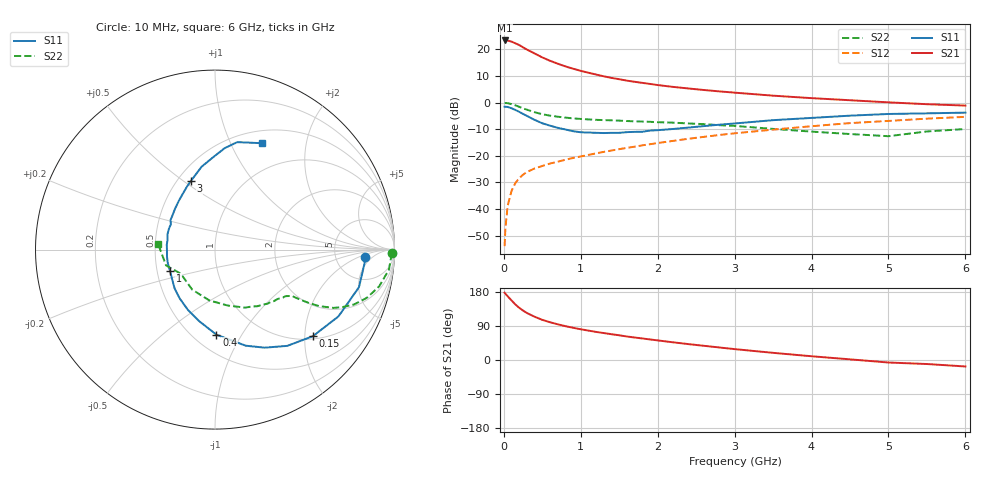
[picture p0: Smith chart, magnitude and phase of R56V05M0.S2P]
! SIEMENS Small Signal Semiconductors
! BFR183
! Si NPN RF Bipolar Junction Transistor in SOT23
! VCE = 6 V  IC = 5 mA
! Common Emitter S-Parameters:  May  1996
# GHz  S  MA  R  50
!  f  S11  S21  S12  S22
! GHz  MAG  ANG  MAG  ANG  MAG  ANG  MAG  ANG
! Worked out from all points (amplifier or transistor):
!   36 points, 10 MHz to 6 GHz, reference 50 ohm
!   highest |S21| = 23.4 dB at 10 MHz (marker M1)
!   |S21| within 3 dB of that: start of sweep to 274.3 MHz
!   unconditionally stable (mu >= 1): 1.052 GHz to 2.66 GHz
!   at 250 MHz: K = 0.42, MSG = 23.9 dB, |S12| = -27.1 dB
!   at 1.4 GHz: K = 1.05, MAG = 12.2 dB, |S12| = -18.0 dB
!   at 6 GHz: K = 0.88, MSG = 2.1 dB, |S12| = -5.4 dB
!   lowest NFmin = 1.15 dB at 450 MHz
!   S11 on the Smith chart (normalised r, x): 10 MHz: 10, -3; 150 MHz: 1.07, -2.20; 400 MHz: 0.64, -0.78; 1 GHz: 0.58, -0.15; 3 GHz: 0.58, +0.53; 6 GHz: 0.65, +1.32
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0.01  0.8377 -2.9  14.73 177.6  0.002 86.8  0.9876 -1.2
0.02  0.8359 -5.7  14.59 175.0  0.0043 83.7  0.982 -2.6
0.05  0.8291 -14.6  14.68 168.1  0.0115 83.2  0.9754 -6.6
0.1  0.7822 -28.4  14.02 157.2  0.0219 76.6  0.9369 -12.7
0.15  0.7281 -41.5  13.01 146.5  0.0308 69.7  0.8877 -17.6
0.2  0.6707 -53.1  12.08 137.8  0.0381 65.5  0.8334 -21.5
0.25  0.6127 -63.1  10.92 130.4  0.0442 61.6  0.7786 -24.3
0.3  0.562 -72.3  9.933 124.0  0.0496 60.1  0.7359 -26.2
0.4  0.4736 -89.1  8.387 114.2  0.0578 57.2  0.6594 -28.5
0.5  0.4086 -102.4  7.065 105.9  0.0644 55.9  0.6042 -29.6
0.6  0.3687 -114.1  6.115 99.7  0.0715 55.9  0.5692 -30.1
0.8  0.3124 -136.0  4.795 89.3  0.0843 56.3  0.5228 -30.8
1  0.2769 -155.1  3.952 81.1  0.0971 57.5  0.493 -31.6
1.1  0.2738 -163.7  3.642 77.6  0.104 58.2  0.4831 -32.4
1.3  0.2677 -178.6  3.119 71.1  0.1185 58.7  0.4684 -33.9
1.6  0.2785 161.4  2.588 62.0  0.141 58.7  0.4505 -37.2
2.2  0.3194 134.0  1.974 46.7  0.1908 57.2  0.4201 -45.8
3  0.4051 109.4  1.539 28.7  0.2647 51.2  0.3649 -62.4
3.5  0.4676 99.2  1.35 18.9  0.3107 45.9  0.3204 -76.9
4.5  0.5681 84.5  1.108 1.7  0.4118 34.3  0.2565 -119.7
5.5  0.628 71.5  0.933 -10.6  0.4992 22.2  0.2868 -162.1
6  0.6481 66.1  0.879 -17.1  0.5399 14.0  0.3188 174.1
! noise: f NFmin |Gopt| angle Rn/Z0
0.45  1.15  0.25  40  0.26
0.9  1.2  0.25  93  0.22
1.8  1.95  0.32  170  0.13
